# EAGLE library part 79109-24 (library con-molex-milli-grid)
RECEPTACAL
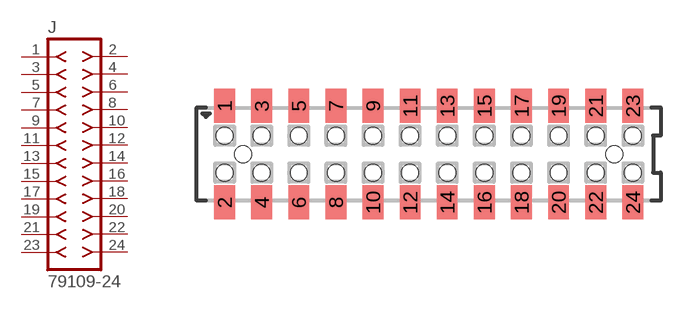
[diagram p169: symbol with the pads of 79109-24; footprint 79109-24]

Designator prefix J

## 79109-24  [79109-24]
1  1  pas
2  2  pas
3  3  pas
4  4  pas
5  5  pas
6  6  pas
7  7  pas
8  8  pas
9  9  pas
10  10  pas
11  11  pas
12  12  pas
13  13  pas
14  14  pas
15  15  pas
16  16  pas
17  17  pas
18  18  pas
19  19  pas
20  20  pas
21  21  pas
22  22  pas
23  23  pas
24  24  pas

## Footprint 79109-24 (pad centres in mm)
RECEPTACAL SMD Dual Row, Vertical, Pass-Thru
smd 1.12 x 1.83: 1 -11,2.6; 2 -11,-2.6; 3 -9,2.6; 4 -9,-2.6; 5 -7,2.6; 6 -7,-2.6; 7 -5,2.6; 8 -5,-2.6; 9 -3,2.6; 10 -3,-2.6; 11 -1,2.6; 12 -1,-2.6; 13 1,2.6; 14 1,-2.6; 15 3,2.6; 16 3,-2.6; 17 5,2.6; 18 5,-2.6; 19 7,2.6; 20 7,-2.6; 21 9,2.6; 22 9,-2.6; 23 11,2.6; 24 11,-2.6
hole 0.914 at -10,0
hole 0.914 at -11,1
hole 0.914 at -11,-1
hole 0.914 at -9,-1
hole 0.914 at -9,1
hole 0.914 at -7,-1
hole 0.914 at -7,1
hole 0.914 at 10,0
hole 0.914 at -5,1
hole 0.914 at -5,-1
hole 0.914 at -3,1
hole 0.914 at -3,-1
hole 0.914 at -1,1
hole 0.914 at -1,-1
hole 0.914 at 1,1
hole 0.914 at 1,-1
hole 0.914 at 3,-1
hole 0.914 at 3,1
hole 0.914 at 5,1
hole 0.914 at 5,-1
hole 0.914 at 7,1
hole 0.914 at 7,-1
hole 0.914 at 9,1
hole 0.914 at 9,-1
hole 0.914 at 11,-1
hole 0.914 at 11,1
